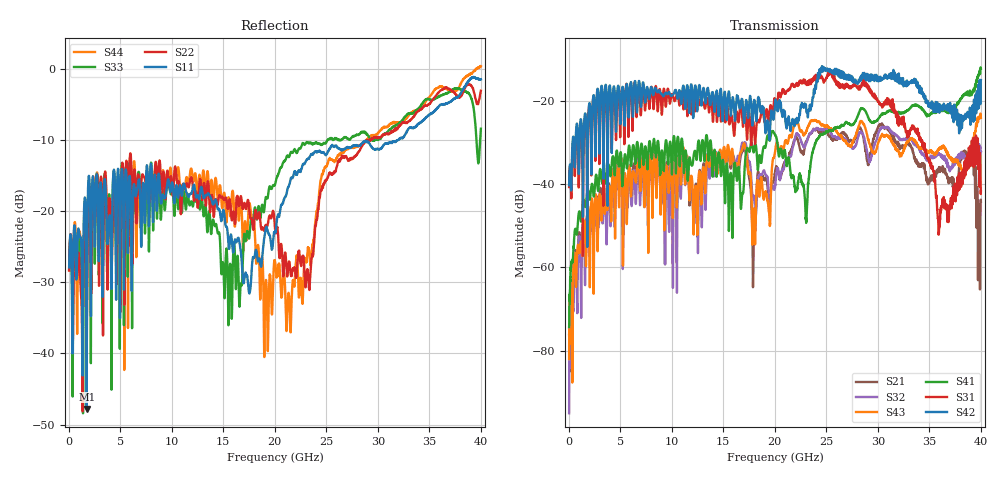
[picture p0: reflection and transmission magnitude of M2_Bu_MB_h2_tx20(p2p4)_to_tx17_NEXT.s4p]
! S11 = S11
! S12 = S12
! S13 = S13
! S14 = S14
! S21 = S21
! S22 = S22
! S23 = S23
! S24 = S24
! S31 = S31
! S32 = S32
! S33 = S33
! S34 = S34
! S41 = S41
! S42 = S42
! S43 = S43
! S44 = S44
! FILE: \\englab.brocade.com\shares\Groups\SIT\Work\Shaohua\IEEE_channels\M2_Bu_MB_h2_tx20(p2p4)_to_tx17_NEXT.s4p
!$DUT_CFG_DESC: Default 4-Port Configuration
!$NUMBER_PORTS: 4
!$DIFF_PORT_MAP: 1|2P|2|2P|0|UC|0|UC|
!$PORT_MAP: PNA 1|1|<<<<<<|TS 2|2|>>>>>>|PNA 2|3|<<<<<<|TS 4|4|>>>>>>|
# MHz S RI R 50.00
! FREQ  S11  S12  S13  S14
!  S21  S22  S23  S24
!  S31  S32  S33  S34
!  S41  S42  S43  S44
!  REAL  IMAG  REAL  IMAG  REAL  IMAG  REAL  IMAG
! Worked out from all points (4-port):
!   3996 points, 50 MHz to 40 GHz, reference 50 ohm
!   strongest paths, dB at 50 MHz, 10.04 GHz, 20.03 GHz, 30.02 GHz, 40 GHz:
!     S42: -40.2, -18.6, -20.8, -14.6, -14.9
!     S31: -40.7, -18.3, -19.6, -20.1, -41.7
!     S41: -74.4, -37.4, -28.2, -24.4, -12.2
!     S43: -82.0, -39.3, -32.3, -30.2, -24.0
!     S32: -95.1, -38.2, -40.3, -27.9, -32.2
!     S21: -76.2, -38.7, -37.1, -26.3, -44.2
!   lowest |S11| = -47.8 dB at 1.76 GHz (marker M1), VSWR 1.01, Z = 49.6 - j0.101 ohm
!   |S11| at or under -10 dB: start of sweep to 31.89 GHz; 31.92722 GHz to 31.96109 GHz (33.87 MHz wide, 0.106 % of centre)
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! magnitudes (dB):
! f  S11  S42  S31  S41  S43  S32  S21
! 50 MHz  -27.9  -40.2  -40.7  -74.4  -82.0  -95.1  -76.2
! 1.76 GHz  -47.8  -30.9  -32.1  -42.8  -50.2  -48.4  -48.2
! 17.98 GHz  -26.5  -20.1  -26.3  -32.1  -46.0  -42.9  -52.3
! 21.42 GHz  -16.2  -25.6  -17.0  -34.5  -28.4  -33.2  -32.6
! 31.28 GHz  -10.4  -14.0  -20.5  -22.3  -29.2  -27.2  -27.9
! 35.94 GHz  -5.2  -21.5  -51.0  -22.4  -31.7  -32.9  -36.7
! 40 GHz  -1.4  -14.9  -41.7  -12.2  -24.0  -32.2  -44.2
